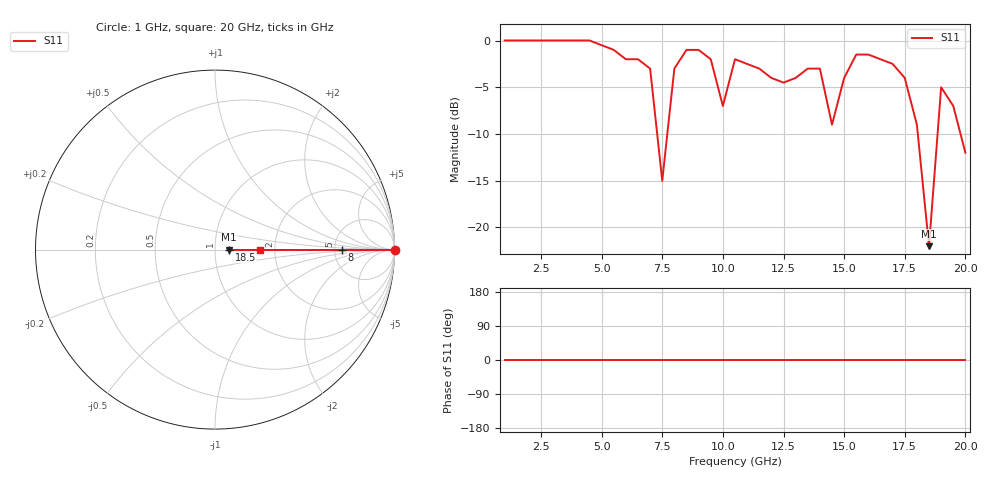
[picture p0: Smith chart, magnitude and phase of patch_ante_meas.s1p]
# GHz S DB R 50
! Generated from TLMsimu/sorre_filter/spara.m based on TLM simulation data
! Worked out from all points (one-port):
!   39 points, 1 GHz to 20 GHz, reference 50 ohm
!   lowest |S11| = -22.0 dB at 18.5 GHz (marker M1), VSWR 1.17, Z = 58.6 + j0 ohm
!   |S11| at or under -10 dB: 7.292 GHz to 7.708 GHz (416.7 MHz wide, 5.56 % of centre); 18.04 GHz to 18.85 GHz (814.5 MHz wide, 4.42 % of centre); 19.8 GHz to end of sweep
!   S11 on the Smith chart (normalised r, x): 1 GHz: open; 8 GHz: 5.85, +0.00; 18.5 GHz: 1.17, +0.00; 20 GHz: 1.67, +0.00
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1  0.01 0.0
3.5  0.01 0.0
4.5  0.01 0.0
6  -2.00 0.0
6.5  -2.00 0.0
7  -3.00 0.0
7.5  -15.00 0.0
8  -3.00 0.0
8.5  -1.00 0.0
9  -1.00 0.0
9.5  -2.00 0.0
10  -7.00 0.0
10.5  -2.00 0.0
12.5  -4.50 0.0
13  -4.00 0.0
13.5  -3.00 0.0
14  -3.00 0.0
14.5  -9.00 0.0
15  -4.00 0.0
15.5  -1.50 0.0
16  -1.50 0.0
17  -2.50 0.0
17.5  -4.00 0.0
18  -9.00 0.0
18.5  -22.00 0.0
19  -5.00 0.0
19.5  -7.00 0.0
20  -12.00 0.0
